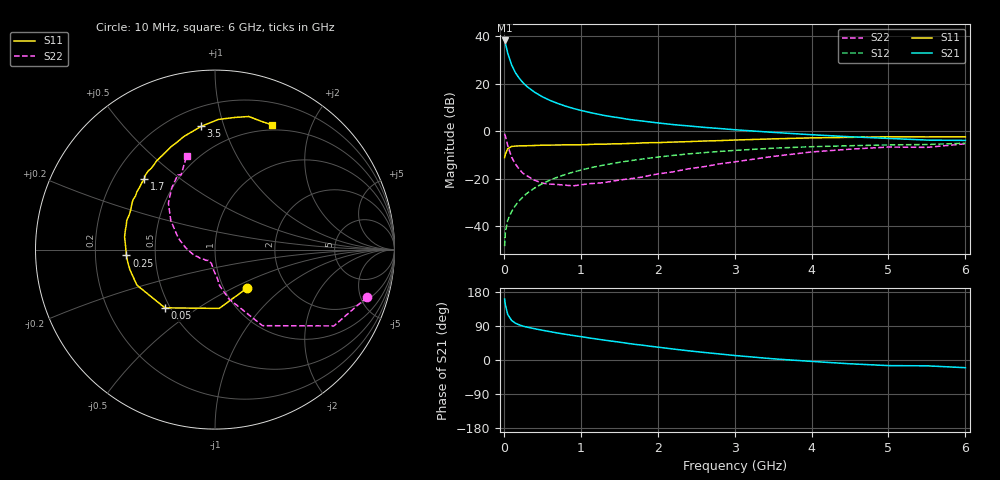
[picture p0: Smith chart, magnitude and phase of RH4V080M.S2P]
! SIEMENS Small Signal Semiconductors
! BFR106
! Si NPN RF Bipolar Junction Transistor in SOT23
! VCE = 4 V  IC = 80 mA
! Common Emitter S-Parameters:  August  1996
# GHz  S  MA  R  50
!  f  S11  S21  S12  S22
! GHz  MAG  ANG  MAG  ANG  MAG  ANG  MAG  ANG
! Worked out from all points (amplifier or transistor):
!   36 points, 10 MHz to 6 GHz, reference 50 ohm
!   highest |S21| = 38.2 dB at 10 MHz (marker M1)
!   |S21| within 3 dB of that: start of sweep to 33.37 MHz
!   unconditionally stable (mu >= 1): 191.3 MHz to 2.423 GHz
!   at 250 MHz: K = 1.05, MAG = 22.7 dB, |S12| = -27.6 dB
!   at 1.4 GHz: K = 1.06, MAG = 8.4 dB, |S12| = -13.7 dB
!   at 6 GHz: K = 0.99, MSG = 0.6 dB, |S12| = -5.0 dB
!   S11 on the Smith chart (normalised r, x): 10 MHz: 1.27, -0.60; 50 MHz: 0.47, -0.37; 250 MHz: 0.34, -0.03; 1.7 GHz: 0.33, +0.37; 3.5 GHz: 0.32, +0.84; 6 GHz: 0.44, +1.46
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0.01  0.2788 -50.9  81.69 160.8  0.0038 79.5  0.887 -17.4
0.02  0.3285 -85.9  71.63 145.8  0.0074 72.3  0.7871 -32.7
0.05  0.428 -130.7  44.33 120.4  0.0133 60.8  0.4998 -58.0
0.1  0.4779 -155.5  25.16 104.6  0.0202 65.3  0.2868 -74.1
0.15  0.487 -166.5  17.17 97.1  0.0273 68.0  0.204 -82.6
0.2  0.4913 -171.8  13.07 92.8  0.0344 70.5  0.1591 -85.5
0.25  0.4944 -176.2  10.48 89.3  0.0416 72.1  0.1296 -90.3
0.3  0.4955 -179.0  8.769 86.8  0.0492 73.0  0.1156 -93.6
0.4  0.5014 175.8  6.642 82.6  0.0639 73.2  0.0929 -99.3
0.5  0.5088 172.0  5.326 78.6  0.0786 73.1  0.0809 -103.8
0.6  0.5108 168.2  4.465 74.8  0.0935 72.5  0.0771 -107.9
0.7  0.5126 164.4  3.856 71.2  0.1082 71.6  0.0755 -113.3
0.9  0.5155 158.1  3.03 64.7  0.1378 68.9  0.0709 -122.0
1.1  0.5262 152.0  2.522 58.5  0.1663 66.3  0.0785 -131.0
1.3  0.534 146.1  2.162 52.6  0.1943 63.2  0.0828 -139.6
1.7  0.5568 135.1  1.715 41.4  0.2472 57.2  0.1028 -156.8
2.2  0.5918 123.3  1.382 29.0  0.31 49.3  0.1398 -175.3
2.8  0.6341 109.6  1.143 16.0  0.3752 39.8  0.2051 164.5
3.5  0.6911 96.4  0.947 3.2  0.4398 29.2  0.2951 146.6
4.5  0.7438 81.7  0.766 -10.0  0.4959 14.5  0.4193 125.1
5.5  0.7599 69.7  0.652 -15.4  0.5263 5.2  0.4574 114.4
6  0.7643 65.6  0.641 -20.3  0.5601 -1.8  0.5451 106.8
